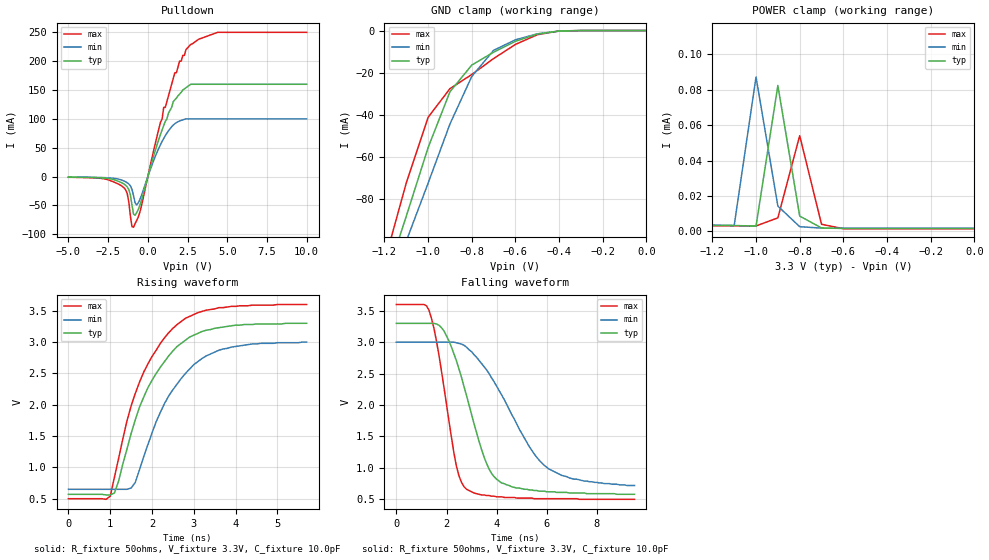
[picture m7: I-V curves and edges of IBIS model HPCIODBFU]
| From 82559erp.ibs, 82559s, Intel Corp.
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[Model]   HPCIODBFU
Model_type   I/O_open_drain
Vinl   =   1.08V   | note : 0.3 * VCCmax
Vinh   =   1.5V   | note : 0.5 * VCCmin
|   typ   min   max
C_comp   2.7pF   NA   NA
| note : on die power/gnd supply distribution R/L/C
|   are not included in the simulation
| note : pull up  mos are not active  pup#="1"
| note : POWER_clamp ref = VIO = VREF = 5.0V
|   variable   typ   min   max
[Voltage range]   3.3V  3.0V   3.6V
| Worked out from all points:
|   slope of the pulldown table from 0 to 0.495 V, typ, clamps not added: 10.4 ohm
|   GND clamp passes 1 mA (typ) near -0.45 V on its own axis
|   POWER clamp passes 1 mA (typ) near -2.35 V on its own axis
|   rising waveform, R_fixture 50ohms, V_fixture 3.3V, C_fixture 10.0pF: 20-80 % time 1.04ns typ, 1.07ns min, 1.01ns max; typ from 0.57 V to 3.3 V
|   falling waveform, R_fixture 50ohms, V_fixture 3.3V, C_fixture 10.0pF: 20-80 % time 1.2ns typ, 1.96ns min, 735ps max; typ from 3.3 V to 0.58 V
| note : all DC curves are with 0.2 OHM res. in series to the PAD.
[GND_clamp]
|Voltage  I(typ)   I(min)   I(max)
-5V       -1.63A     -1.47A     -1.85A
-1.2V     -120mA     -130mA     -110mA
-1.1V     -88.2mA    -100mA     -72.4mA
-1V       -55.6mA    -72.5mA    -41.2mA
-900mV    -29.1mA    -44.4mA    -27.6mA
-800mV    -16.4mA    -21.8mA    -20.9mA
-700mV    -10.3mA    -9.39mA    -13.3mA
-600mV    -5.12mA    -4.42mA    -6.6mA
-500mV    -1.67mA    -1.57mA    -2mA
-400mV    -240uA     -300uA     -220uA
0V        0A         0A         0A
[PullDown]
|Voltage   I(typ)   I(min)   I(max)
-5V       -970uA     -730uA     -1.18mA
-1.6V     -11.3mA    -6.5mA     -17.1mA
-1.2V     -22.3mA    -12.7mA    -43.8mA
-1V       -49.2mA    -21.8mA    -86.7mA
-900mV    -65mA      -33.2mA    -87.6mA
-800mV    -66.9mA    -45.7mA    -81.4mA
-600mV    -56.9mA    -45.4mA    -69.8mA
1V        88.6mA     66.1mA     120mA
1.6V      130mA      89.2mA     170mA
2.4V      154mA      100mA      220mA
4.4V      160mA      100mA      250mA
10V       160mA      100mA      250mA
[POWER_clamp]
|Voltage   I(typ)   I(min)   I(max)
-5V       11.6A      10.3A      12.9A
-2.6V     230mA      830uA      1.23A
-2.4V     1.77mA     6.84uA     400mA
-2.2V     6.3uA      4.14uA     5.23mA
-2.1V     4.05uA     4.05uA     120uA
-2V       3.88uA     3.97uA     5.85uA
-1.1V     3.35uA     3.39uA     3.15uA
-1V       3.04uA     87.1uA     3.11uA
-900mV    82.3uA     14.3uA     7.67uA
-800mV    8.69uA     2.7uA      54uA
-700mV    1.98uA     1.89uA     4.06uA
0V        1.65uA     1.83uA     1.47uA
[Ramp]
| note : pad parasitics are not included
|Variable   typ   min   max
dV/dt_r   1.64/0.4n   1.41/0.5n   1.86/0.4n
dV/dt_f   1.63/1.2n   1.37/2.0n   1.86/0.7n
| note : 50ohms RES. always connected to VCC
R_load =   50ohms
[Rising Waveform]
| note : pad parasitics are not included
| note : input changes at T=0.5nS
| note : input data is to vox_data
R_fixture   = 50ohms
V_fixture   = 3.3V
V_fixture_min   = 3.0V
V_fixture_max   = 3.6V
C_fixture   = 10.0pF
| note : the 50ohms RES. is connected to VCC
|Time   typ(V)  min(V)  max(V)
0s        570mV      650mV      500mV
1ns       560mV      650mV      540mV
1.2ns     780mV      650mV      1.14V
1.5ns     1.54V      670mV      1.98V
1.7ns     1.96V      960mV      2.36V
2.1ns     2.5V       1.73V      2.87V
2.6ns     2.93V      2.33V      3.28V
3ns       3.11V      2.64V      3.44V
3.6ns     3.23V      2.87V      3.55V
5.7ns     3.3V       3V         3.6V
[Falling Waveform]
| note : pad parasitics are not included
| note : input changes at T=0.5nS
| note : input data is to vox_data
R_fixture   = 50ohms
V_fixture   = 3.3V
V_fixture_min   = 3.0V
V_fixture_max   = 3.6V
C_fixture   = 10.0pF
|Time   typ   min   max
0s        3.3V       3V         3.6V
1.3ns     3.3V       3V         3.51V
1.9ns     3.18V      3V         2.28V
2.4ns     2.7V       2.99V      1.02V
2.8ns     2.15V      2.92V      660mV
3.6ns     1.07V      2.56V      560mV
4.2ns     760mV      2.16V      540mV
5.3ns     650mV      1.34V      520mV
6.1ns     620mV      980mV      510mV
9.5ns     580mV      720mV      500mV
